(* Logix 5000 AddOnInstructionDefinition export P2M2HBVL_P2HL_AB_BNI00E1_PD_R0; software revision 31.00 *)

TYPE IO_Link_Port_Data :
STRUCT
   Inputs : SINT[48];
   Outputs : SINT[48];
END_STRUCT
END_TYPE

TYPE UDT_P2M2HBVL_P2HL_ProcData :
STRUCT
   Status : UDT_P2M2HBVL_P2HL_Process_Inputs;
   EV : UDT_P2M2HBVL_P2HL_Process_Outputs;
END_STRUCT
END_TYPE

TYPE UDT_P2M2HBVL_P2HL_Process_Inputs :
STRUCT
   Fail_Safe : BOOL;
   Aux_Volt_Warning : BOOL;
   Aux_Volt_Failure : BOOL;
   Module_Failure : BOOL;
   Module_Over_Temp : BOOL;
   Module_Over_Load : BOOL;
   Short_Circuit : BOOL;
   Output_Stage_Not_Available : BOOL;
   Device_OK : BOOL;
   Mismatch_Fault : BOOL;
   Comm_Fault : BOOL;
   Validation_Failed : BOOL;
   Event_1_Error_Code : SINT;
   Event_1_Add_Code_1 : SINT;
   Event_1_Add_Code_2 : SINT;
   Event_2_Error_Code : SINT;
   Event_2_Add_Code_1 : SINT;
   Event_2_Add_Code_2 : SINT;
   Event_3_Error_Code : SINT;
   Event_3_Add_Code_1 : SINT;
   Event_3_Add_Code_2 : SINT;
END_STRUCT
END_TYPE

TYPE UDT_P2M2HBVL_P2HL_Process_Outputs :
STRUCT
   _01 : BOOL;   // EV1 Command
   _02 : BOOL;   // EV2 Command
   _03 : BOOL;   // EV3 Command
   _04 : BOOL;   // EV4 Command
   _05 : BOOL;   // EV5 Command
   _06 : BOOL;   // EV6 Command
   _07 : BOOL;   // EV7 Command
   _08 : BOOL;   // EV8 Command
   _09 : BOOL;   // EV9 Command
   _10 : BOOL;   // EV10 Command
   _11 : BOOL;   // EV11 Command
   _12 : BOOL;   // EV12 Command
   _13 : BOOL;   // EV13 Command
   _14 : BOOL;   // EV14 Command
   _15 : BOOL;   // EV15 Command
   _16 : BOOL;   // EV16 Command
   _17 : BOOL;   // EV17 Command
   _18 : BOOL;   // EV18 Command
   _19 : BOOL;   // EV19 Command
   _20 : BOOL;   // EV20 Command
   _21 : BOOL;   // EV21 Command
   _22 : BOOL;   // EV22 Command
   _23 : BOOL;   // EV23 Command
   _24 : BOOL;   // EV24 Command
END_STRUCT
END_TYPE

ADD_ON_INSTRUCTION P2M2HBVL_P2HL_AB_BNI00E1_PD_R0   (* revision 3.0, vendor Parker-Hannifin Corp. *)
// Parker P2M or P2H IO-Link
// Firmware rev >= 1.10
// with Balluff BNI00E1
// IO-Link Master
// Revision note:
// 9/29/2017 Initial release
// 5/14/2018 Limit cycle count, Add system cmd
// 5/24/2018 Separated PD and PRN
// 2/7/2019 Revised to accomodate P2H IOL
VAR_IN_OUT
   Balluff_Port_Data : IO_Link_Port_Data; {required}
        .INPUTS[0].0   // Read Diagnostic Bit 0 From Port
        .INPUTS[0].1   // Read Diagnostic Bit 1 From Port
        .INPUTS[0].2   // Read Diagnostic Bit 2 From Port
        .INPUTS[0].3   // Read Diagnostic Bit 3 From Port
        .INPUTS[0].4   // Read Diagnostic Bit 4 From Port
        .INPUTS[0].5   // Read Diagnostic Bit 5 From Port
        .INPUTS[0].6   // Read Diagnostic Bit 6 From Port
        .INPUTS[0].7   // Read Diagnostic Bit 7 From Port
        .INPUTS[32].0   // Port in IO-Link Mode
        .INPUTS[32].1   // Slave Device Connected
        .INPUTS[33].0   // Device Validation Failed
        .INPUTS[34]   // Vendor ID (high byte)
        .INPUTS[35]   // Vendor ID (low byte)
        .INPUTS[36]   // Device ID (high byte)
        .INPUTS[37]   // Device ID (middle byte)
        .INPUTS[38]   // Device ID (low byte)
        .OUTPUTS[0].0   // Send EV1 Command to Port
        .OUTPUTS[0].1   // Send EV2 Command to Port
        .OUTPUTS[0].2   // Send EV3 Command to Port
        .OUTPUTS[0].3   // Send EV4 Command to Port
        .OUTPUTS[0].4   // Send EV5 Command to Port
        .OUTPUTS[0].5   // Send EV6 Command to Port
        .OUTPUTS[0].6   // Send EV7 Command to Port
        .OUTPUTS[0].7   // Send EV8 Command to Port
        .OUTPUTS[1].0   // Send EV9 Command to Port
        .OUTPUTS[1].1   // Send EV10 Command to Port
        .OUTPUTS[1].2   // Send EV11 Command to Port
        .OUTPUTS[1].3   // Send EV12 Command to Port
        .OUTPUTS[1].4   // Send EV13 Command to Port
        .OUTPUTS[1].5   // Send EV14 Command to Port
        .OUTPUTS[1].6   // Send EV15 Command to Port
        .OUTPUTS[1].7   // Send EV16 Command to Port
        .OUTPUTS[2].0   // Send EV17 Command to Port
        .OUTPUTS[2].1   // Send EV18 Command to Port
        .OUTPUTS[2].2   // Send EV19 Command to Port
        .OUTPUTS[2].3   // Send EV20 Command to Port
        .OUTPUTS[2].4   // Send EV21 Command to Port
        .OUTPUTS[2].5   // Send EV22 Command to Port
        .OUTPUTS[2].6   // Send EV23 Command to Port
        .OUTPUTS[2].7   // Send EV24 Command to Port
   Data : UDT_P2M2HBVL_P2HL_ProcData; {required}
END_VAR

ROUTINE Logic   (* ladder *)
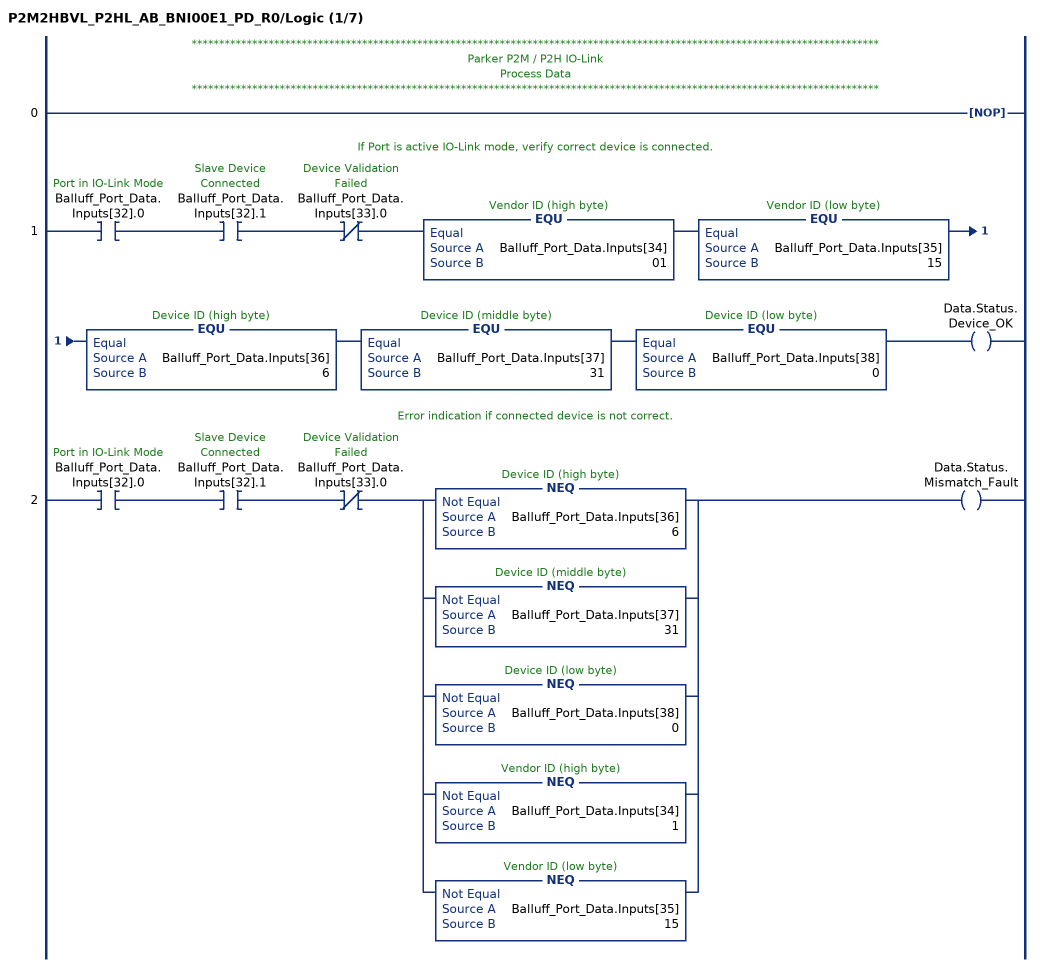
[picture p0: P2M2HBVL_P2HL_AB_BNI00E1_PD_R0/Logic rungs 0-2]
   // *****************************************************************************************************************************
   // Parker P2M / P2H IO-Link
   // Process Data
   // *****************************************************************************************************************************
   0: NOP();
   // If Port is active IO-Link mode, verify correct device is connected.
   1: XIC(Balluff_Port_Data.Inputs[32].0)XIC(Balluff_Port_Data.Inputs[32].1)XIO(Balluff_Port_Data.Inputs[33].0)EQU(Balluff_Port_Data.Inputs[34],01)EQU(Balluff_Port_Data.Inputs[35],15)EQU(Balluff_Port_Data.Inputs[36],6)EQU(Balluff_Port_Data.Inputs[37],31)EQU(Balluff_Port_Data.Inputs[38],0)OTE(Data.Status.Device_OK);
   // Error indication if connected device is not correct.
   2: XIC(Balluff_Port_Data.Inputs[32].0)XIC(Balluff_Port_Data.Inputs[32].1)XIO(Balluff_Port_Data.Inputs[33].0)[NEQ(Balluff_Port_Data.Inputs[36],6) ,NEQ(Balluff_Port_Data.Inputs[37],31) ,NEQ(Balluff_Port_Data.Inputs[38],0) ,NEQ(Balluff_Port_Data.Inputs[34],1) ,NEQ(Balluff_Port_Data.Inputs[35],15) ]OTE(Data.Status.Mismatch_Fault);
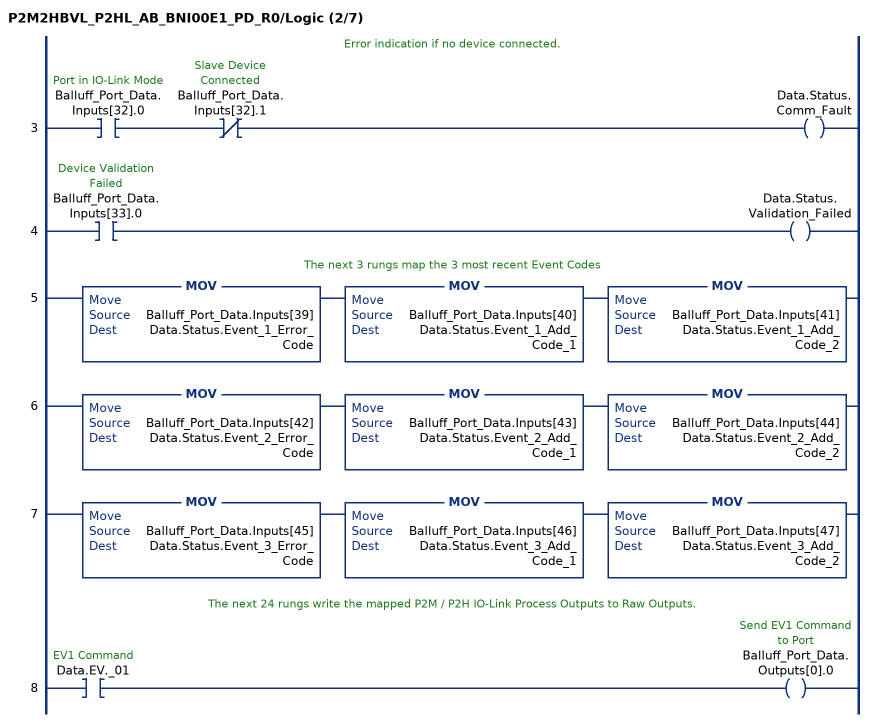
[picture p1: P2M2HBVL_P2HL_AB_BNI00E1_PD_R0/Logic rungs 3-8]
   // Error indication if no device connected.
   3: XIC(Balluff_Port_Data.Inputs[32].0)XIO(Balluff_Port_Data.Inputs[32].1)OTE(Data.Status.Comm_Fault);
   4: XIC(Balluff_Port_Data.Inputs[33].0)OTE(Data.Status.Validation_Failed);
   // The next 3 rungs map the 3 most recent Event Codes
   5: MOV(Balluff_Port_Data.Inputs[39],Data.Status.Event_1_Error_Code)MOV(Balluff_Port_Data.Inputs[40],Data.Status.Event_1_Add_Code_1)MOV(Balluff_Port_Data.Inputs[41],Data.Status.Event_1_Add_Code_2);
   6: MOV(Balluff_Port_Data.Inputs[42],Data.Status.Event_2_Error_Code)MOV(Balluff_Port_Data.Inputs[43],Data.Status.Event_2_Add_Code_1)MOV(Balluff_Port_Data.Inputs[44],Data.Status.Event_2_Add_Code_2);
   7: MOV(Balluff_Port_Data.Inputs[45],Data.Status.Event_3_Error_Code)MOV(Balluff_Port_Data.Inputs[46],Data.Status.Event_3_Add_Code_1)MOV(Balluff_Port_Data.Inputs[47],Data.Status.Event_3_Add_Code_2);
   // The next 24 rungs write the mapped P2M / P2H IO-Link Process Outputs to Raw Outputs.
   8: XIC(Data.EV._01)OTE(Balluff_Port_Data.Outputs[0].0);
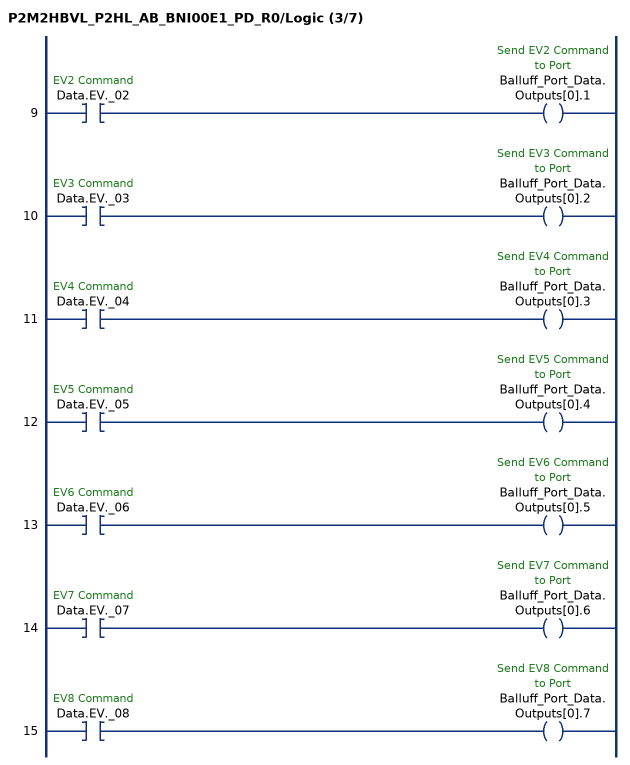
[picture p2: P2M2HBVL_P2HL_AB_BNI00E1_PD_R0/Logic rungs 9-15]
   9: XIC(Data.EV._02)OTE(Balluff_Port_Data.Outputs[0].1);
   10: XIC(Data.EV._03)OTE(Balluff_Port_Data.Outputs[0].2);
   11: XIC(Data.EV._04)OTE(Balluff_Port_Data.Outputs[0].3);
   12: XIC(Data.EV._05)OTE(Balluff_Port_Data.Outputs[0].4);
   13: XIC(Data.EV._06)OTE(Balluff_Port_Data.Outputs[0].5);
   14: XIC(Data.EV._07)OTE(Balluff_Port_Data.Outputs[0].6);
   15: XIC(Data.EV._08)OTE(Balluff_Port_Data.Outputs[0].7);
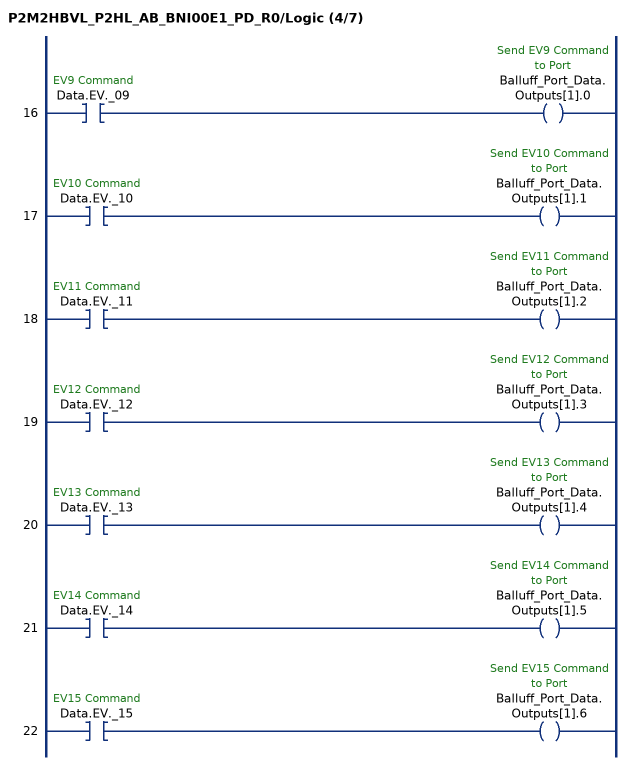
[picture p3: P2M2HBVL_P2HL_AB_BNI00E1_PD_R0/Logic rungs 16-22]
   16: XIC(Data.EV._09)OTE(Balluff_Port_Data.Outputs[1].0);
   17: XIC(Data.EV._10)OTE(Balluff_Port_Data.Outputs[1].1);
   18: XIC(Data.EV._11)OTE(Balluff_Port_Data.Outputs[1].2);
   19: XIC(Data.EV._12)OTE(Balluff_Port_Data.Outputs[1].3);
   20: XIC(Data.EV._13)OTE(Balluff_Port_Data.Outputs[1].4);
   21: XIC(Data.EV._14)OTE(Balluff_Port_Data.Outputs[1].5);
   22: XIC(Data.EV._15)OTE(Balluff_Port_Data.Outputs[1].6);
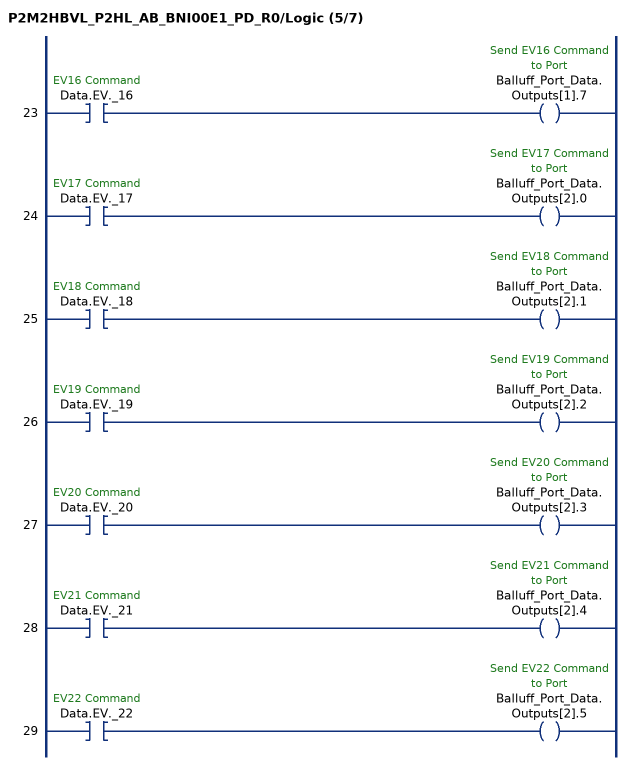
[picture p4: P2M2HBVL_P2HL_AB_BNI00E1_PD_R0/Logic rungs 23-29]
   23: XIC(Data.EV._16)OTE(Balluff_Port_Data.Outputs[1].7);
   24: XIC(Data.EV._17)OTE(Balluff_Port_Data.Outputs[2].0);
   25: XIC(Data.EV._18)OTE(Balluff_Port_Data.Outputs[2].1);
   26: XIC(Data.EV._19)OTE(Balluff_Port_Data.Outputs[2].2);
   27: XIC(Data.EV._20)OTE(Balluff_Port_Data.Outputs[2].3);
   28: XIC(Data.EV._21)OTE(Balluff_Port_Data.Outputs[2].4);
   29: XIC(Data.EV._22)OTE(Balluff_Port_Data.Outputs[2].5);
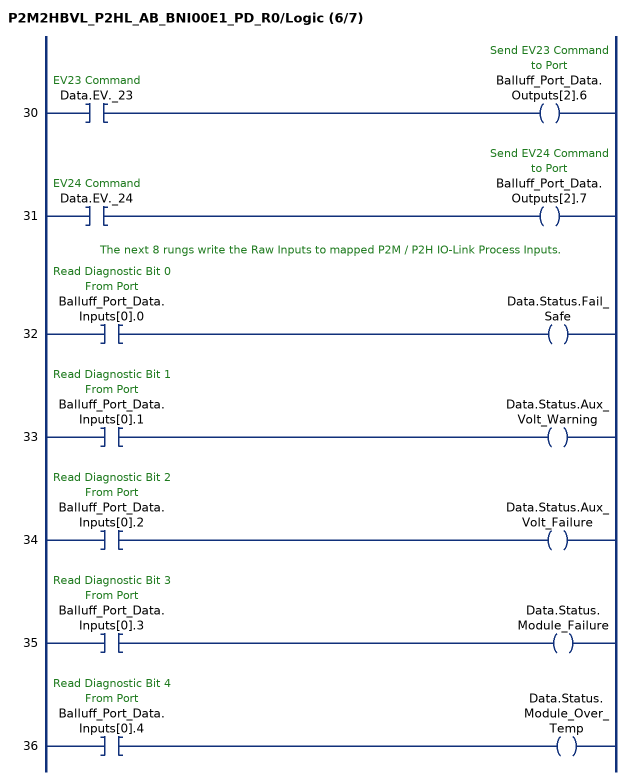
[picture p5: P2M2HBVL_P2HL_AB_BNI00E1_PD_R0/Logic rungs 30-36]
   30: XIC(Data.EV._23)OTE(Balluff_Port_Data.Outputs[2].6);
   31: XIC(Data.EV._24)OTE(Balluff_Port_Data.Outputs[2].7);
   // The next 8 rungs write the Raw Inputs to mapped P2M / P2H IO-Link Process Inputs.
   32: XIC(Balluff_Port_Data.Inputs[0].0)OTE(Data.Status.Fail_Safe);
   33: XIC(Balluff_Port_Data.Inputs[0].1)OTE(Data.Status.Aux_Volt_Warning);
   34: XIC(Balluff_Port_Data.Inputs[0].2)OTE(Data.Status.Aux_Volt_Failure);
   35: XIC(Balluff_Port_Data.Inputs[0].3)OTE(Data.Status.Module_Failure);
   36: XIC(Balluff_Port_Data.Inputs[0].4)OTE(Data.Status.Module_Over_Temp);
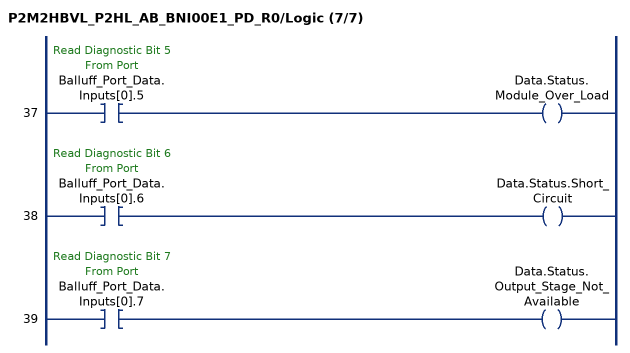
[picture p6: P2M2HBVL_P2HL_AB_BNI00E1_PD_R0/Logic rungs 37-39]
   37: XIC(Balluff_Port_Data.Inputs[0].5)OTE(Data.Status.Module_Over_Load);
   38: XIC(Balluff_Port_Data.Inputs[0].6)OTE(Data.Status.Short_Circuit);
   39: XIC(Balluff_Port_Data.Inputs[0].7)OTE(Data.Status.Output_Stage_Not_Available);
END_ROUTINE
END_ADD_ON_INSTRUCTION
